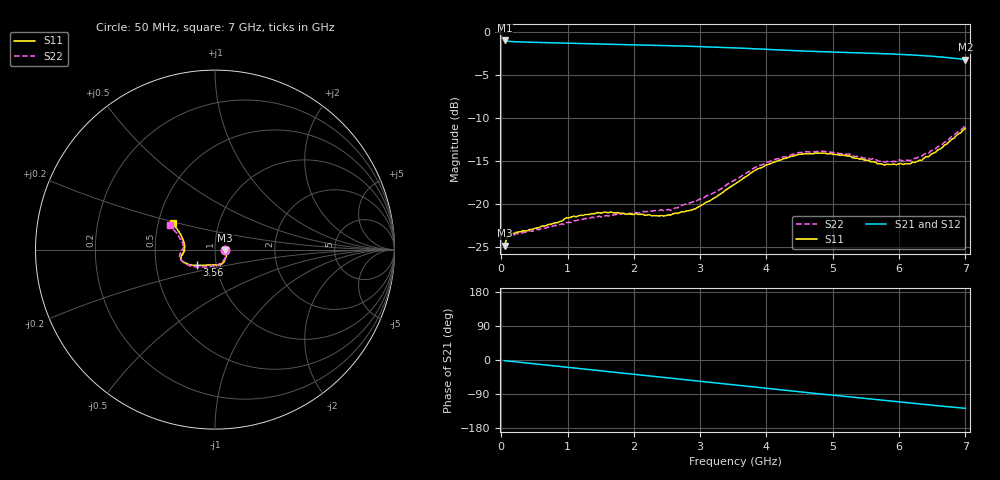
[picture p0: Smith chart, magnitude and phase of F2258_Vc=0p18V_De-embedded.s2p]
! Integrated Device Technology
! Corporate Headquarters
! 6024 Silver Creek Valley Road
! San Jose, CA 95138  USA
! Phone:  1-408-284-8200
! Toll Free:  1-800-223-1366
! Webpage:  http://www.idt.com/
! Timing and RF Division
! 515 Groton Road, Suite 102
! Westford, MA 01886-6024
! Device:  F2258
! Description: Voltage Variable RF Attenuator
! Frequency:  50.0 -  6000.00 MHz
! Package:  3x3 mm Thin QFN Plastic Package: 16 pin
! Ports:  2 RF, 2 DC
!  Pin  1  = NC
!  Pin  2  = NC
!  Pin  3  = RF2  = Port 2
!  Pin  4  = GND
!  Pin  5  = Vdd
!  Pin  6  = NC
!  Pin  7  = VCTRL
!  Pin  8  = NC
!  Pin  9  = GND
!  Pin 10  = RF1  = Port 1
!  Pin 11  = NC
!  Pin 12  = NC
!  Pin 13  = NC
!  Pin 14  = NC
!  Pin 15  = NC
!  Pin 16  = NC
! Vcntrl:  0.180 Volts
! Vdd:  +3.300 Volts
! Current:  1.077 mA
! Data:  The device was measured on a the F2258 evaluation board which has
!  individual transmission lines to the RF pins.  Data was collected
!  using a calibrated network analyzer.  The evaluation board was
!  de-embedded using a TRL calibration technique.
!  The reference plane is the edge of the package pin.
! Misc:  SN 10
!  Action Tracker AT0285
! Date Measured:  2014-12-10
! Date:  2016-01-13  MJV
! Note:
!  Integrated Device Technology supplies this data as a sample of measured
!  data at the package pin for this product.  Your particular data for this
!  product may vary.
!  Data was taken at 25 degrees C.
!  Integrated Device Technology reserves the right to change this data at anytime.
!Freq_(GHz)  S11M_(dB)  S11P_(deg)  S21M_(dB)  S21P_(deg)  S12M_(dB)  S12P_(deg)  S22M_(dB)  S22P_(deg)
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# GHz S dB R 50
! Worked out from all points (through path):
!   201 points, 50 MHz to 7 GHz, reference 50 ohm
!   highest |S21| = -0.96 dB at 50 MHz (marker M1); lowest = -3.2 dB at 7 GHz (marker M2)
!   group delay of S21, straight-line fit = 50.5 ps
!   lowest |S11| = -24.9 dB at 50 MHz (marker M3), VSWR 1.12, Z = 56 - j0.39 ohm
!   |S11| at or under -10 dB: start of sweep to end of sweep
!   |S22| runs from -24.9 to -10.9 dB; largest |S21 - S12| = 0.00041
!   S11 on the Smith chart (normalised r, x): 50 MHz: 1.12, -0.01; 3.56 GHz: 0.81, -0.14; 7 GHz: 0.60, +0.19
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0.05  -24.88 -3.5  -0.96 -1.9  -0.96 -1.9  -24.93 -3.0
0.08475  -23.91 -5.9  -1.03 -2.4  -1.03 -2.4  -23.98 -5.5
0.15425  -23.42 -9.3  -1.08 -3.6  -1.08 -3.6  -23.60 -9.4
0.71025  -22.39 -37.2  -1.22 -14.1  -1.22 -14.1  -22.69 -38.6
0.98825  -21.61 -51.1  -1.27 -19.3  -1.27 -19.3  -22.17 -54.7
1.2315  -21.35 -59.3  -1.32 -23.8  -1.32 -23.8  -21.80 -63.7
1.6485  -20.95 -71.0  -1.41 -31.4  -1.41 -31.4  -21.31 -76.7
2.37825  -21.41 -92.5  -1.54 -44.8  -1.54 -44.8  -20.78 -94.3
2.552  -21.31 -98.4  -1.57 -48.0  -1.57 -48.0  -20.74 -99.6
2.93425  -20.54 -115.1  -1.65 -55.1  -1.65 -55.1  -19.73 -113.0
3.525  -17.69 -137.8  -1.82 -66.2  -1.82 -66.2  -17.21 -135.6
3.55975  -17.50 -138.8  -1.83 -66.9  -1.83 -66.9  -17.03 -136.6
4.0115  -15.42 -151.4  -2.00 -75.2  -2.00 -75.2  -15.12 -151.0
4.46325  -14.28 -159.8  -2.16 -83.4  -2.16 -83.4  -14.07 -162.1
4.7065  -14.15 -163.0  -2.23 -87.7  -2.23 -87.7  -13.96 -166.3
5.2625  -14.42 -170.0  -2.38 -97.4  -2.38 -97.4  -14.21 -174.3
5.6795  -15.35 -176.8  -2.46 -104.6  -2.47 -104.6  -15.03 -179.7
5.85325  -15.41 179.0  -2.52 -107.8  -2.52 -107.8  -15.06 175.7
6.166  -15.34 171.2  -2.63 -113.4  -2.63 -113.4  -14.97 169.8
6.33975  -14.93 164.9  -2.71 -116.5  -2.71 -116.5  -14.43 165.4
6.722  -13.01 153.3  -2.94 -123.1  -2.94 -123.1  -12.71 156.4
7  -11.19 147.9  -3.19 -127.4  -3.19 -127.4  -10.92 151.4
